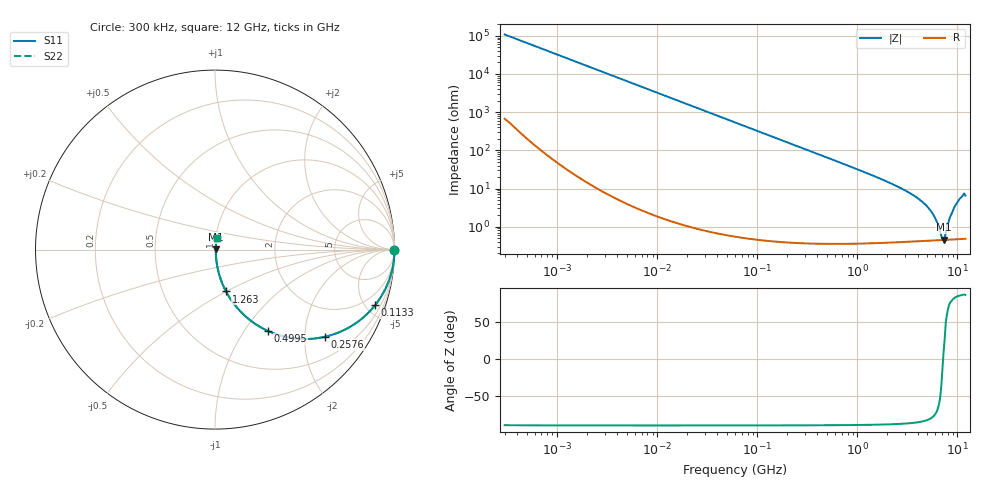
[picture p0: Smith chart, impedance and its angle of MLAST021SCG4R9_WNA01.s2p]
! MLAST021SCG4R9_WNA01  S-PARAMETER MODEL  ( General Type )
! Model Generated by TAIYO YUDEN Corporation (http://www.ty-top.com)
! Version 1.0
! TAIYO YUDEN Control No. 220901
! Copyright(c) 2022 TAIYO YUDEN CO.,LTD. All Rights Reserved.
! Product Description (link to TY-COMPAS)
! https://ds.yuden.co.jp/TYCOMPAS/or/detail?pn=MLAST021SCG4R9BWNA01&u=M
! Products Name : Multilayer Ceramic Capacitors
! Characteristics :
!  Capacitance : 4.9 pF , Rated Voltage : 25V , TCC : CG / C0G
!  Case Size : 0.25 x 0.125 / 0.0098 x 0.0049 [mm/inch] , Thickness : 0.125 / 0.0049 [mm/inch]
!  (Conditions: Temperature = 25 degC , DC Bias Current/Voltage = 0A / 0V)
! External Node Assignments :
!  1  o---| |---o  2
! GND o---------o GND
! Frequency Range : 0.3MHz  -  12000MHz  [ 401 STEP ]
# MHz S RI R 50
! Freq[MHz].  S11 Real  S11 Imag  S21 Real  S21 Imag  S12 Real  S12 Imag  S22 Real  S22 Imag
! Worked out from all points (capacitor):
!   401 points, 300 kHz to 12 GHz, reference 50 ohm
!   read as one part in series: C = 4.9 pF near 316.3 kHz
!   lowest |Z| = 454 mohm at 7.254 GHz (marker M1)
!   series resonance near 7.192 GHz, so ESL is about 100 pH
!   S11 on the Smith chart (normalised r, x): 300 kHz: open; 113.3 MHz: 1.01, -5.73; 257.6 MHz: 1.01, -2.52; 499.5 MHz: 1.01, -1.29; 1.263 GHz: 1.01, -0.50; 12 GHz: 1.01, +0.13
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0.3  1 -0.000924  6.56e-06 0.000924  6.56e-06 0.000924  1 -0.000924
1.769972  1 -0.00545  3.49e-05 0.00545  3.49e-05 0.00545  1 -0.00545
10.44266  0.9989 -0.0321  0.00105 0.0321  0.00105 0.0321  0.9989 -0.0321
60  0.9668 -0.1786  0.0332 0.1786  0.0332 0.1786  0.9668 -0.1786
113.3117  0.8911 -0.3108  0.1089 0.3108  0.1089 0.3108  0.8911 -0.3108
168.5979  0.7871 -0.4083  0.2129 0.4083  0.2129 0.4083  0.7871 -0.4083
257.5933  0.613 -0.4856  0.387 0.4856  0.387 0.4856  0.613 -0.4856
353.9943  0.456 -0.4961  0.544 0.4961  0.544 0.4961  0.456 -0.4961
499.5319  0.2961 -0.4538  0.7039 0.4538  0.7039 0.4538  0.2961 -0.4538
783.7017  0.1458 -0.3486  0.8542 0.3486  0.8542 0.3486  0.1458 -0.3486
1262.535  0.0615 -0.2331  0.9385 0.2331  0.9385 0.2331  0.0615 -0.2331
2088.533  0.0234 -0.1384  0.9766 0.1384  0.9766 0.1384  0.0234 -0.1384
3454.93  0.00916 -0.0711  0.9908 0.0711  0.9908 0.0711  0.00916 -0.0711
4875.354  0.0055 -0.0354  0.9945 0.0354  0.9945 0.0354  0.0055 -0.0354
5868.704  0.00468 -0.018  0.9953 0.018  0.9953 0.018  0.00468 -0.018
6879.757  0.00447 -0.00354  0.9955 0.00354  0.9955 0.00354  0.00447 -0.00354
7254.098  0.00449 0.000565  0.9955 -0.000565  0.9955 -0.000565  0.00449 0.000565
7648.807  0.00454 0.00519  0.9955 -0.00519  0.9955 -0.00519  0.00454 0.00519
8503.825  0.00491 0.018  0.9951 -0.018  0.9951 -0.018  0.00491 0.018
9454.42  0.00583 0.0342  0.9942 -0.0342  0.9942 -0.0342  0.00583 0.0342
11083.22  0.00846 0.0607  0.9915 -0.0607  0.9915 -0.0607  0.00846 0.0607
12000  0.00891 0.0638  0.9911 -0.0638  0.9911 -0.0638  0.00891 0.0638
